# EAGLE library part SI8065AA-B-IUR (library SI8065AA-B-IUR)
Digital Isolators 6 ch 1 kV digital isolator Source: Datasheet
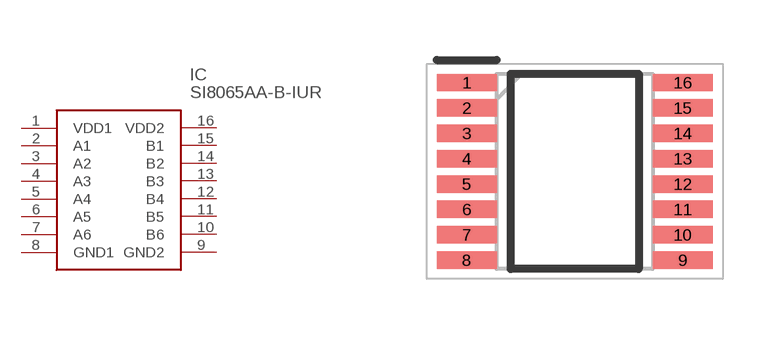
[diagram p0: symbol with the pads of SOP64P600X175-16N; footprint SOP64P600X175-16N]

Designator prefix IC

## SI8065AA-B-IUR (Description: Digital Isolators 6 ch 1 kV digital isolator; Height: 1.75mm; Manufacturer_Name: Skyworks; Manufacturer_Part_Number: SI8065AA-B-IUR; Mouser_Part_Number: 634-SI8065AA-B-IUR; Mouser_Price-Stock: https://www.mouser.co.uk/ProductDetail/Skyworks-Solutions-Inc/SI8065AA-B-IUR?qs=j6MGy4L9yX0oMTeiOOvMHA%3D%3D)  [SOP64P600X175-16N]
1  VDD1
2  A1
3  A2
4  A3
5  A4
6  A5
7  A6
8  GND1
9  GND2
10  B6
11  B5
12  B4
13  B3
14  B2
15  B1
16  VDD2

## Footprint SOP64P600X175-16N (pad centres in mm)
SI8065AA-B-IUR*
smd 1.5 x 0.435: 1 -2.7,2.222; 2 -2.7,1.588; 3 -2.7,0.952; 4 -2.7,0.318; 5 -2.7,-0.318; 6 -2.7,-0.952; 7 -2.7,-1.588; 8 -2.7,-2.222; 9 2.7,-2.222; 10 2.7,-1.588; 11 2.7,-0.952; 12 2.7,-0.318; 13 2.7,0.318; 14 2.7,0.952; 15 2.7,1.588; 16 2.7,2.222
